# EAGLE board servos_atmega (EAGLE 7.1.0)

Size 100 x 80 mm. Coordinates in mm from the lower left corner, seen from the top.
Outline: 0,0 100,0 100,80 0,80 0,0
Copper layers (1*16): Top 0.035mm / dielectric 1.5mm / Bottom 0.035mm
Design rules "default": minimum track width 10mil, minimum drill 24mil, track to track 8mil, track to pad 8mil, pad to pad 8mil, via to via 8mil, smd to smd 8mil, copper to edge 40mil, drill to drill 8mil, minimum pad ring 10mil, minimum via ring 8mil, stop-mask expansion 4mil, vias tented up to drill 0mil, thermal gap 10mil

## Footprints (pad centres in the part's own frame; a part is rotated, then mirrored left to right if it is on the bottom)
0402-CAP = smd 0.7 x 0.9: 1 -0.65,0; 2 0.65,0
TC26V = drill 0.813: 1 -1.27,0; 2 1.27,0
0402-RES = smd 0.7 x 0.9: 1 -0.65,0; 2 0.65,0
MA03-1 = drill 1.016 long: 1 -2.54,0; 2 0,0; 3 2.54,0
MLF32-PAD = smd 0.7 x 0.3: 1 -2.35,1.75; 2 -2.35,1.25; 3 -2.35,0.75; 4 -2.35,0.25; 5 -2.35,-0.25; 6 -2.35,-0.75; 7 -2.35,-1.25; 8 -2.35,-1.75; 17 2.35,-1.75; 18 2.35,-1.25; 19 2.35,-0.75; 20 2.35,-0.25; 21 2.35,0.25; 22 2.35,0.75; 23 2.35,1.25; 24 2.35,1.75 | smd 0.3 x 0.7: 9 -1.75,-2.35; 10 -1.25,-2.35; 11 -0.75,-2.35; 12 -0.25,-2.35; 13 0.25,-2.35; 14 0.75,-2.35; 15 1.25,-2.35; 16 1.75,-2.35; 25 1.75,2.35; 26 1.25,2.35; 27 0.75,2.35; 28 0.25,2.35; 29 -0.25,2.35; 30 -0.75,2.35; 31 -1.25,2.35; 32 -1.75,2.35 | smd 3.2 x 3.2: PAD 0,0

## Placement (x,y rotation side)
C1  22pf  [0402-CAP]  91.44,78.74 180 top
C2  22pf  [0402-CAP]  87.63,78.74 180 top
CRYSTAL  16MHz  [TC26V]  85.09,60.96 0 top
R1  1k  [0402-RES]  95.25,72.39 270 top
R2  1k  [0402-RES]  81.28,71.12 270 top
R3  1k  [0402-RES]  77.47,72.39 270 top
R4  1k  [0402-RES]  73.66,71.12 270 top
R5  1k  [0402-RES]  71.12,69.85 270 top
RPUP  10k  [0402-RES]  90.17,62.23 180 top
SV1  [MA03-1]  66.04,78.74 180 top
SV2  [MA03-1]  73.66,78.74 180 top
SV3  [MA03-1]  81.28,78.74 180 top
SV4  [MA03-1]  97.79,59.69 90 top
SV5  [MA03-1]  97.79,72.39 90 top
U1  [MLF32-PAD]  87.63,69.85 270 top

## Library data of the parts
C1 C2 R1-R5 RPUP = SparkFun-Passives
CRYSTAL = crystal; OC_FARNELL: unknown; OC_NEWARK: unknown
SV1-SV5 = con-lstb; OC_FARNELL: unknown; OC_NEWARK: unknown
U1 = SparkFun-DigitalIC

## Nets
GND: C1.2 C2.2 CRYSTAL.1 CRYSTAL.2 SV1.1 SV2.1 SV3.1 SV4.1 SV5.1 U1.3 U1.5 U1.21 U1.PAD
N$1: R5.2 U1.15
N$2: R4.2 U1.14
N$3: R3.2 U1.13
N$4: RPUP.1 U1.29
N$5: R2.1 SV4.2
N$6: R1.1 SV5.2
N$7: R2.2 U1.10
N$8: R1.2 U1.9
N$9: R3.1 SV3.2
N$10: C1.1 U1.8
N$11: C2.1 U1.7
N$12: R5.1 SV1.2
N$13: R4.1 SV2.2
VCC: RPUP.2 SV1.3 SV2.3 SV3.3 SV4.3 SV5.3 U1.4 U1.6 U1.18

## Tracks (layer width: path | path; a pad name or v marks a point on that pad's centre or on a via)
GND  (12 unrouted)
N$1  (1 unrouted)
N$2  (1 unrouted)
N$3  (1 unrouted)
N$4  (1 unrouted)
N$5  (1 unrouted)
N$6  (1 unrouted)
N$7  (1 unrouted)
N$8  (1 unrouted)
N$9  (1 unrouted)
N$10  (1 unrouted)
N$11  (1 unrouted)
N$12  (1 unrouted)
N$13  (1 unrouted)
VCC  (8 unrouted)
